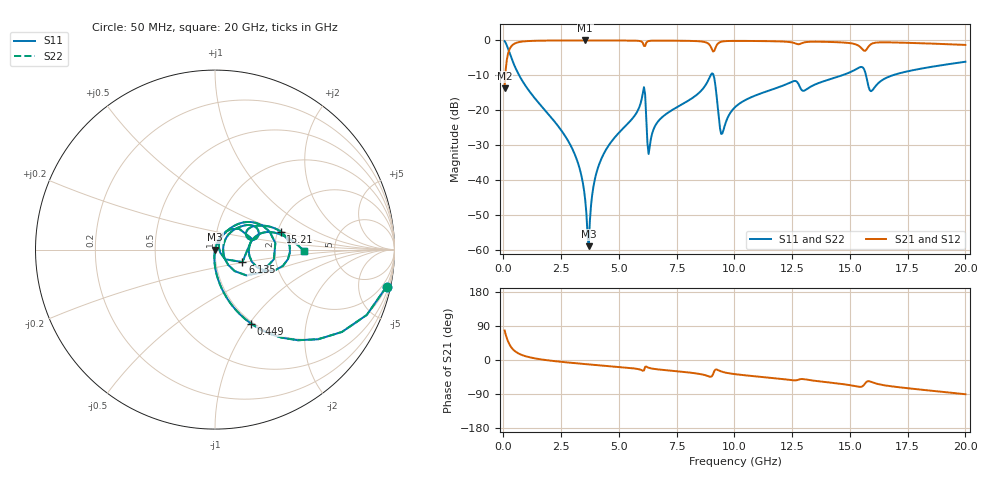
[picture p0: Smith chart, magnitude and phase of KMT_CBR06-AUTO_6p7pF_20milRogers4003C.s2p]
! Data measured by Modelithics Inc. support@modelithics.com 813-866-6335
! KEMET CBR06-AUTO 6.7pF, Pad Width= 0.851mm, Pad Length= 0.64mm, Pad Gap= 0.62mm, 20mil Rogers 4003C substrate Data, January 2022
# hz S ma R 50
! 2 Port Network Data from SP1.SP block
! freq  magS11  angS11  magS21  angS21  magS12  angS12  magS22  angS22
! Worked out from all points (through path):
!   401 points, 50 MHz to 20 GHz, reference 50 ohm
!   highest |S21| = -0.01 dB at 3.541 GHz (marker M1); lowest = -13.6 dB at 50 MHz (marker M2)
!   group delay of S21, straight-line fit = 14 ps
!   lowest |S11| = -58.8 dB at 3.691 GHz (marker M3), VSWR 1.00, Z = 50.1 + j0.0323 ohm
!   |S11| at or under -10 dB: 683 MHz to 8.968 GHz (8.285 GHz wide, 172 % of centre); 9.096 GHz to 14.65 GHz (5.553 GHz wide, 46.8 % of centre); 15.7 GHz to 16.84 GHz (1.139 GHz wide, 7 % of centre)
!   |S22| runs from -58.8 to -0.2 dB; largest |S21 - S12| = 0
!   S11 on the Smith chart (normalised r, x): 50 MHz: 0.98, -9.29; 449 MHz: 0.98, -1.02; 6.135 GHz: 1.34, -0.19; 15.21 GHz: 2.08, +0.49; 20 GHz: 2.96, -0.07
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5e7  0.9781 -12.2  0.2079 77.8  0.2079 77.8  0.9781 -12.2
2.495e8  0.6843 -47.6  0.7287 42.4  0.7287 42.4  0.6843 -47.6
4.49e8  0.4589 -64.0  0.8879 25.9  0.8879 25.9  0.4589 -64.0
2.74325e9  0.03946 -95.0  0.9982 -6.3  0.9982 -6.3  0.03946 -95.0
3.391625e9  0.01103 -94.9  0.9989 -10.0  0.9989 -10.0  0.01103 -94.9
3.54125e9  0.00523 -89.8  0.9989 -10.8  0.9989 -10.8  0.00523 -89.8
3.690875e9  0.001149 16.3  0.9989 -11.6  0.9989 -11.6  0.001149 16.3
3.94025e9  0.009747 70.9  0.9988 -12.9  0.9988 -12.9  0.009747 70.9
4.289375e9  0.02215 72.4  0.9985 -14.7  0.9985 -14.7  0.02215 72.4
6.035e9  0.1774 41.1  0.9236 -28.4  0.9236 -28.4  0.1774 41.1
6.13475e9  0.1677 -24.5  0.8329 -18.0  0.8329 -18.0  0.1677 -24.5
6.33425e9  0.03081 44.3  0.9867 -21.3  0.9867 -21.3  0.03081 44.3
6.73325e9  0.07213 62.2  0.9938 -25.1  0.9938 -25.1  0.07213 62.2
9.0275e9  0.3381 6.2  0.7445 -42.7  0.7445 -42.7  0.3381 6.2
9.4265e9  0.04607 -8.5  0.9567 -30.2  0.9567 -30.2  0.04607 -8.5
1.0025e10  0.1111 48.1  0.9846 -37.4  0.9846 -37.4  0.1111 48.1
1.336662e10  0.2243 32.0  0.9586 -54.0  0.9586 -54.0  0.2243 32.0
1.5212e10  0.3791 15.3  0.8859 -68.7  0.8859 -68.7  0.3791 15.3
1.556112e10  0.4102 -7.4  0.7353 -68.7  0.7353 -68.7  0.4102 -7.4
1.591025e10  0.1883 -1.6  0.8817 -57.6  0.8817 -57.6  0.1883 -1.6
1.670825e10  0.3052 18.7  0.9378 -68.7  0.9378 -68.7  0.3052 18.7
2e10  0.4957 -1.0  0.8619 -90.3  0.8619 -90.3  0.4957 -1.0
